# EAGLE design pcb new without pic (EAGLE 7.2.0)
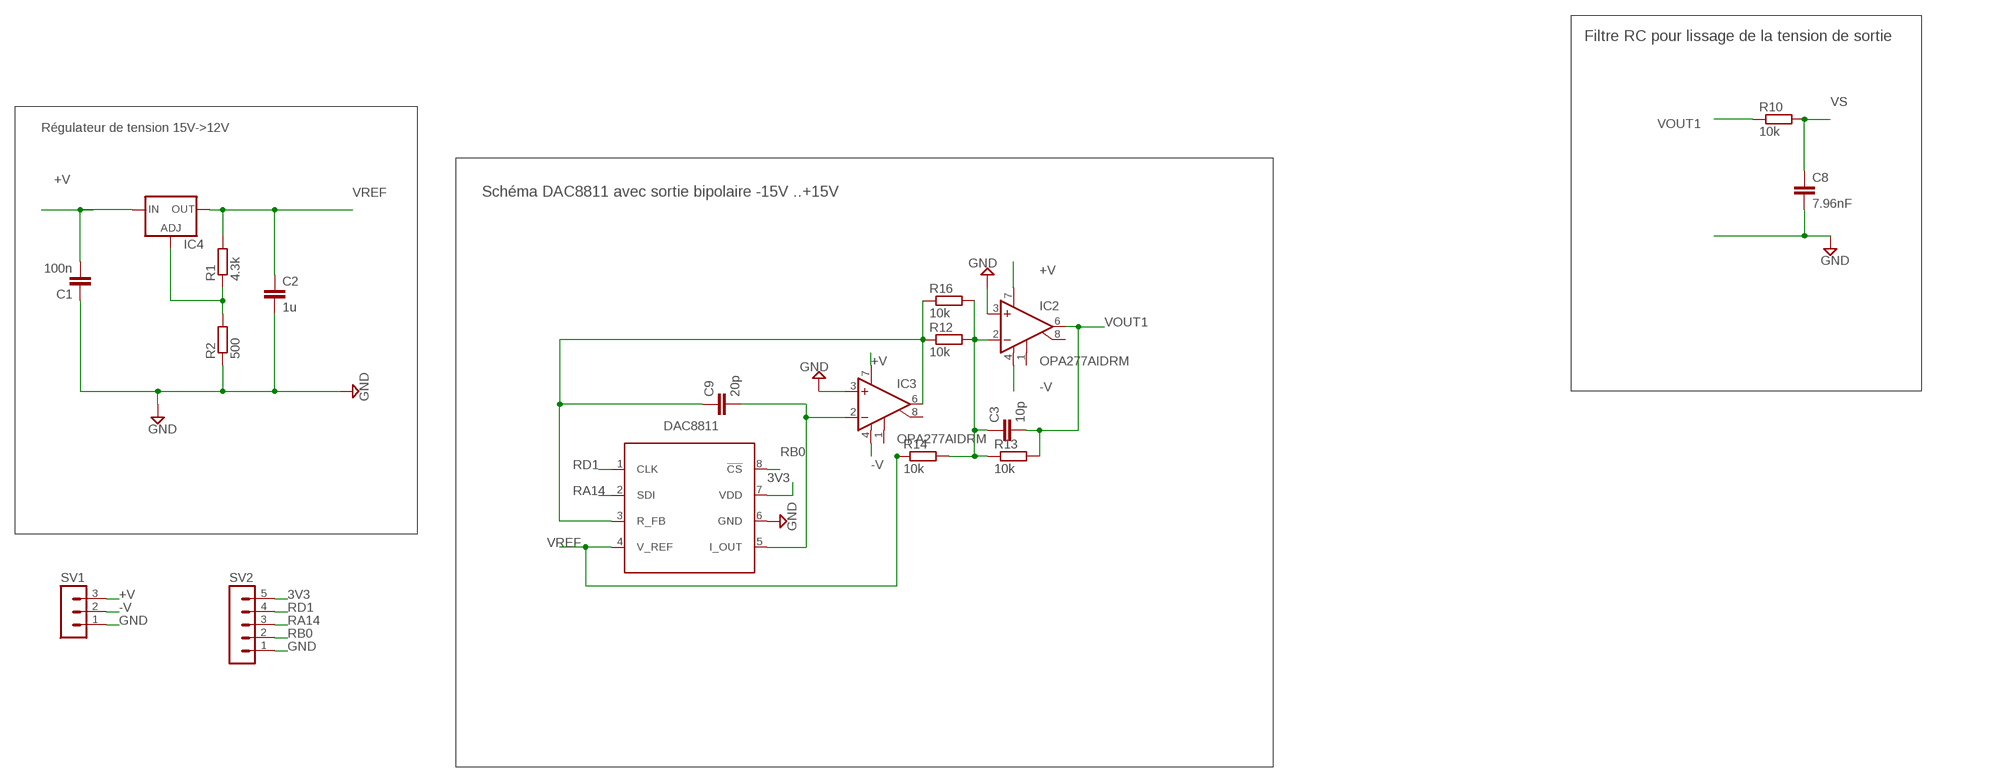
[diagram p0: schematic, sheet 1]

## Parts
C1  100n  C-EUC0603  [C0603]
C2  1u  C-EUC0603  [C0603]
C3  10p  C-EUC0603  [C0603]
C8  7.96nF  C-EUC0603  [C0603]
C9  20p  C-EUC0603  [C0603]
DAC8811  DAC8811  [DAC8811]
IC2  OPA277AIDRM  [DFN8-4X4]
IC3  OPA277AIDRM  [DFN8-4X4]
IC4  LM317-T039  [TO39-H03]
R1  4.3k  R-EU_R0603  [R0603]
R2  500  R-EU_R0603  [R0603]
R10  10k  R-EU_R0603  [R0603]
R12  10k  R-EU_R0805  [R0805]
R13  10k  R-EU_R0805  [R0805]
R14  10k  R-EU_R0805  [R0805]
R16  10k  R-EU_R0805  [R0805]
SV1  MA03-1  [MA03-1]
SV2  MA05-1  [MA05-1]

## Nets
3V3: DAC8811.7(VDD) SV2.5
+V: C1.2 IC2.7(V+) IC3.7(V+) IC4.1(IN) SV1.3
-V: IC2.4(V-) IC3.4(V-) SV1.2
GND: C1.1 C2.2 C8.2 DAC8811.6(GND) IC2.3(+IN) IC3.3(+IN) R2.1 SV1.1 SV2.1
I_OUT: C9.2 DAC8811.5(I_OUT) IC3.2(-IN)
N$1: IC4.2(ADJ) R1.1 R2.2
N$6: C3.1 IC2.2(-IN) R12.2 R13.1 R14.2 R16.2
R_FB: C9.1 DAC8811.3(R_FB) IC3.6(OUT) R12.1 R16.1
RA14: DAC8811.2(SDI) SV2.3
RB0: DAC8811.8(!CS) SV2.2
RD1: DAC8811.1(CLK) SV2.4
VOUT1: C3.2 IC2.6(OUT) R10.1 R13.2
VREF: C2.1 DAC8811.4(V_REF) IC4.3(OUT) R1.2 R14.1
VS: C8.1 R10.2
Unconnected: IC2.1(CMP1) IC2.8(CMP2) IC3.1(CMP1) IC3.8(CMP2)

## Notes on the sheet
- Filtre RC pour lissage de la tension de sortie
- Régulateur de tension 15V->12V
- Schéma DAC8811 avec sortie bipolaire -15V ..+15V

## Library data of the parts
C1-C3 C8 C9 = resistor:C-EU: CAPACITOR, European symbol
DAC8811 = dac:DAC8811
IC2 IC3 = linear:OPA277: High Precision OPERATIONAL AMPLIFIERS REPLACES OP-07, OP-77, OP-177 Source: opa277.pdf
IC4 = v-reg:LM317-T039: VOLTAGE REGULATOR
R1 R2 R10 R12-R14 R16 = resistor:R-EU_: RESISTOR, European symbol
SV1 = con-lstb:MA03-1: PIN HEADER; OC_FARNELL: unknown; OC_NEWARK: unknown
SV2 = con-lstb:MA05-1: PIN HEADER; OC_FARNELL: unknown; OC_NEWARK: unknown

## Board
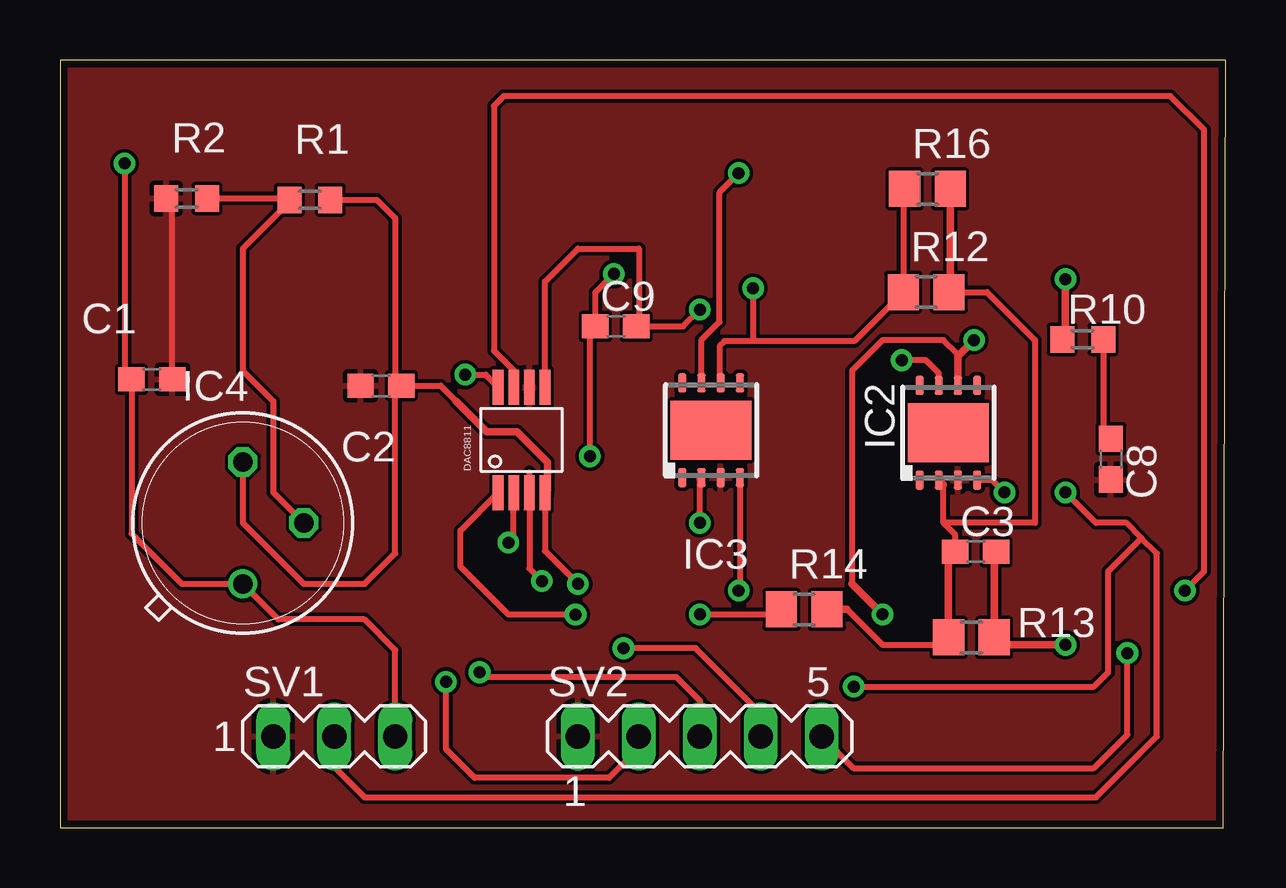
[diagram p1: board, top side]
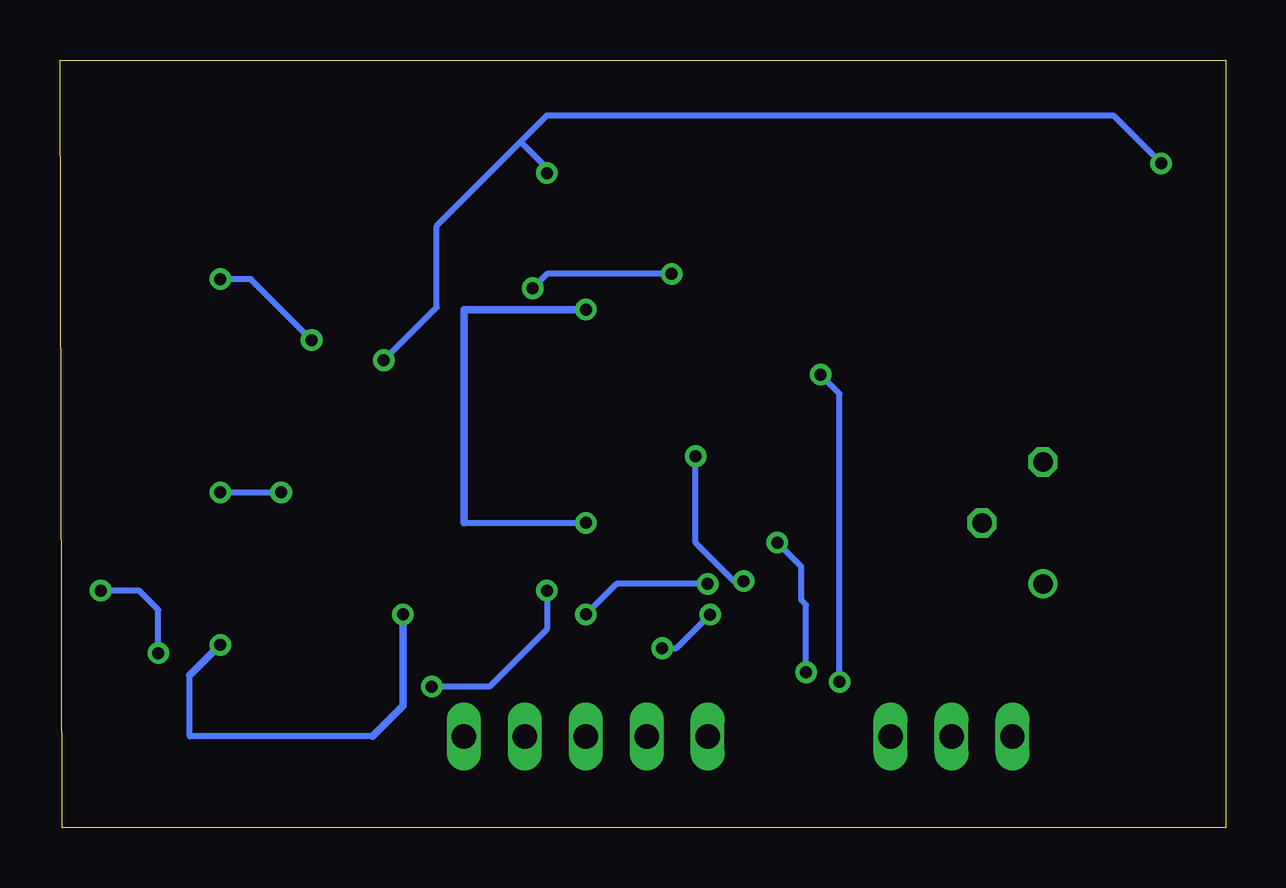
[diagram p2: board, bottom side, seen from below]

Size 48.59 x 31.99 mm. Coordinates in mm from the lower left corner, seen from the top.
Outline: 0,0 48.49,0 48.59,31.99 0,31.99 0,0
Copper layers (1*16): Top 0.035mm / dielectric 1.5mm / Bottom 0.035mm
Design rules "default *": minimum track width 0.15mm, minimum drill 0.3mm, track to track 0.15mm, track to pad 0.15mm, pad to pad 0.15mm, via to via 0.15mm, smd to smd 0.15mm, copper to edge 0.3mm, drill to drill 0.2mm, minimum pad ring 0.2mm, minimum via ring 0.15mm, stop-mask expansion 0.075mm, vias tented up to drill 0mil, thermal gap 0.2mm

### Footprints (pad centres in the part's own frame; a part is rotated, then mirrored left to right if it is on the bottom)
C0603 = smd 1.1 x 1: 1 -0.85,0; 2 0.85,0
DAC8811 = smd 0.45 x 1.45: 1 -0.975,-2.2; 2 -0.325,-2.2; 3 0.325,-2.2; 4 0.975,-2.2; 5 0.975,2.2; 6 0.325,2.2; 7 -0.325,2.2; 8 -0.975,2.2
DFN8-4X4 = smd 0.35 x 0.8: 1 -1.2,-1.975; 2 -0.4,-1.975; 3 0.4,-1.975; 4 1.2,-1.975; 5 1.2,1.975; 6 0.4,1.975; 7 -0.4,1.975; 8 -1.2,1.975 | smd 3.38 x 2.45: TH 0,0
TO39-H03 = drill 0.813: 1 0,-2.54 | drill 0.813 octagon: 2 2.54,0; 3 0,2.54
R0603 = smd 1 x 1.1: 1 -0.85,0; 2 0.85,0
R0805 = smd 1.3 x 1.5: 1 -0.95,0; 2 0.95,0
MA03-1 = drill 1.016 long: 1 -2.54,0; 2 0,0; 3 2.54,0
MA05-1 = drill 1.016 long: 1 -5.08,0; 2 -2.54,0; 3 0,0; 4 2.54,0; 5 5.08,0

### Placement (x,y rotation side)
C1  3.83,18.68 180 top
C2  13.38,18.42 180 top
C3  38.17,11.5 0 top
C8  43.81,15.36 270 top
C9  23.17,20.89 0 top
DAC8811  19.24,16.16 0 top
IC2  37.03,16.46 0 top
IC3  27.14,16.56 0 top
IC4  7.62,12.7 0 top
R1  10.41,26.16 0 top
R2  5.28,26.22 0 top
R10  42.63,20.35 0 top
R12  36.1,22.32 0 top
R13  37.99,7.93 0 top
R14  31.02,9.1 0 top
R16  36.16,26.62 0 top
SV1  11.43,3.81 0 top
SV2  26.67,3.81 0 top

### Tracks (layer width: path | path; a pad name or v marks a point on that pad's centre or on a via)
3V3  (via drill 0.5)
  Top 0.254: SV2.5 33.08,2.48 43.09,2.48 44.49,3.88 v44.49,7.28 | v46.89,9.88 47.69,10.68 47.69,29.08 46.29,30.48 18.49,30.48 18.09,30.08 18.09,19.88 18.91,19.05 DAC8811.7
  Bottom 0.254: v44.49,7.28 44.49,9.08 45.29,9.88 v46.89,9.88
+V  (via drill 0.5)
  Top 0.254: IC2.7 36.63,18.94 36.09,19.48 v35.09,19.48 | v2.69,27.68 2.69,18.97 C1.2 2.98,12.26 5.08,10.16 IC4.1 9.1,8.68 12.69,8.68 13.97,7.4 SV1.3 | IC3.7 26.74,20.33 27.49,21.08 27.49,26.48 v28.29,27.28
  Bottom 0.254: v35.09,19.48 32.89,21.68 32.89,25.08 29.39,28.58 | 29.39,28.58 28.29,29.68 4.69,29.68 v2.69,27.68 | v28.29,27.28 28.29,27.48 29.39,28.58
-V  (via drill 0.5)
  Top 0.254: SV1.2 11.43,2.54 12.7,1.27 43.18,1.27 45.72,3.81 45.72,11.43 45.08,12.07 | 45.08,12.07 44.45,12.7 43.18,12.7 v41.91,13.97 | v39.37,13.97 38.86,14.48 IC2.4 | IC3.4 28.34,9.93 v28.29,9.88 | v33.09,5.88 43.09,5.88 43.69,6.48 43.69,10.68 45.08,12.07
  Bottom 0.254: v41.91,13.97 v39.37,13.97 | v28.29,9.88 28.29,8.28 30.69,5.88 v33.09,5.88
GND
  Top 0.254: C1.1 4.68,25.97 R2.1
  pour Top: -1.27,32.82 49.53,33.02 49.53,-1.27 -1.27,-1.27
I_OUT  (via drill 0.5)
  Top 0.254: DAC8811.5 20.21,22.76 21.59,24.13 24.13,24.13 24.13,21 | C9.2 25.97,20.89 v26.67,21.59 | v26.67,12.7 26.67,14.52
  Top 0.305: 24.13,21 C9.2 | 26.67,14.52 IC3.2
  Bottom 0.254: 31.75,12.7 v26.67,12.7
  Bottom 0.305: v26.67,21.59 31.75,21.59 31.75,12.7
N$1
  Top 0.254: R2.2 9.51,26.22 R1.1 9.56,26.07 7.62,24.13 7.62,19.05 8.89,17.78 8.89,13.97 IC4.2
N$6
  Top 0.254: R12.2 38.64,22.32 40.64,20.32 40.64,12.7 36.83,12.7 | 36.83,12.7 36.83,14.28 | 32.81,9.1 34.29,7.62 36.73,7.62 | C3.1 37.32,12.21 36.83,12.7
  Top 0.305: R16.2 37.11,22.38 R12.2 | 36.83,14.28 IC2.2 | R14.2 32.81,9.1 | 36.73,7.62 R13.1 37.04,11.22 C3.1
R_FB  (via drill 0.5)
  Top 0.254: R16.1 35.15,26.56 R12.1 33.11,20.28 28.89,20.28 | 28.89,20.28 27.69,20.28 27.49,20.08 27.49,18.59 IC3.6 | v23.09,23.08 22.32,22.31 C9.1 22.09,20.66 v22.09,15.48 | v28.89,22.48 28.89,20.28 | DAC8811.3 19.49,13.88 | DAC8811.3 19.57,14.8 | DAC8811.3 19.57,10.8 v20.09,10.28
  Bottom 0.254: v23.09,23.08 28.29,23.08 v28.89,22.48 | v20.09,10.28 20.49,10.28 22.09,11.88 v22.09,15.48
RA14  (via drill 0.5)
  Top 0.254: 26.16,3.81 SV2.3 26.67,5.3 25.69,6.28 17.69,6.28 v17.49,6.48 | v18.69,11.88 18.91,12.1 DAC8811.2
  Bottom 0.254: v17.49,6.48 17.49,9.28 17.69,9.48 17.69,10.88 v18.69,11.88
RB0  (via drill 0.5)
  Top 0.254: SV2.2 24.13,3.32 22.89,2.08 17.29,2.08 16.09,3.28 v16.09,6.08 | v16.89,18.88 17.75,18.88 DAC8811.8
  Bottom 0.254: v16.09,6.08 16.09,18.08 v16.89,18.88
RD1  (via drill 0.5)
  Top 0.254: SV2.4 29.21,4.76 26.49,7.48 v23.49,7.48 | v21.49,8.88 18.69,8.88 16.69,10.88 16.69,12.38 DAC8811.1
  Bottom 0.254: v23.49,7.48 22.89,7.48 v21.49,8.88
VOUT1  (via drill 0.5)
  Top 0.254: IC2.6 37.43,19.72 36.83,20.32 34.29,20.32 33.02,19.05 33.02,10.16
  Top 0.305: IC2.6 37.43,19.65 v38.1,20.32 | v41.91,22.86 41.91,20.48 R10.1 | C3.2 38.94,11.42 R13.2 39.25,7.62 v41.91,7.62 | 33.02,10.16 v34.29,8.89
  Bottom 0.254: v38.1,20.32 40.64,22.86 v41.91,22.86 | 35.56,3.81 43.18,3.81 43.18,6.35
  Bottom 0.305: v34.29,8.89 34.29,5.08 35.56,3.81 | 43.18,6.35 v41.91,7.62
VREF  (via drill 0.5)
  Top 0.254: IC4.3 7.62,12.7 10.16,10.16 12.7,10.16 13.97,11.43 13.97,18.16 | R1.2 13.21,26.16 13.97,25.4 13.97,18.68 | C2.1 15.87,18.42 16.51,17.78 | 20.32,13.85 DAC8811.4 20.21,11.54 v21.59,10.16 | v26.67,8.89 29.86,8.89
  Top 0.305: 13.97,18.16 C2.1 13.97,18.68 | 29.86,8.89 R14.1 | 16.51,17.78 17.78,16.51 19.05,16.51 20.32,15.24 20.32,14.06 DAC8811.4
  Bottom 0.254: v21.59,10.16 25.4,10.16 v26.67,8.89
VS
  Top 0.254: R10.2 43.48,16.54
  Top 0.305: 43.48,16.54 C8.1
